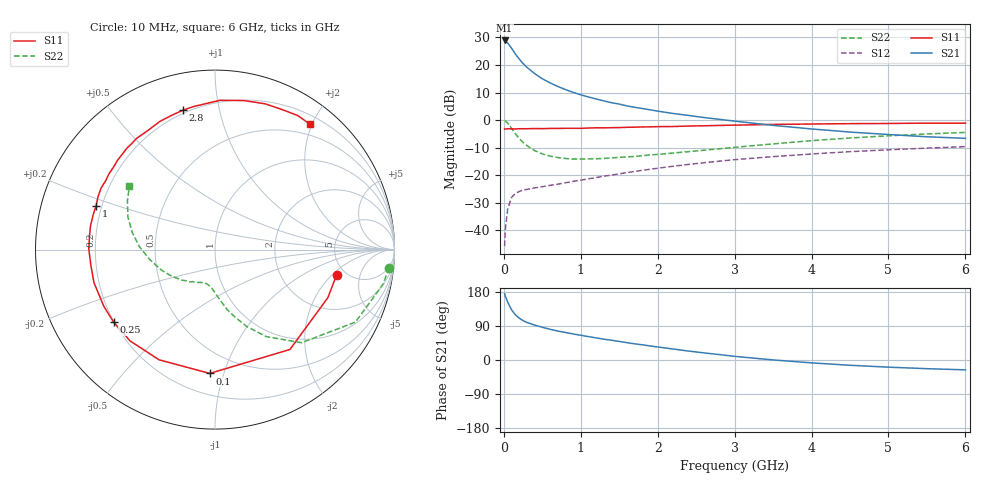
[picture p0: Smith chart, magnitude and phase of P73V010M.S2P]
! SIEMENS Small Signal Semiconductors
! BFP196
! Si NPN RF Bipolar Junction Transistor in SOT143
! VCE = 3 V  IC = 10 mA
! Common Emitter S-Parameters:  May  1996
# GHz  S  MA  R  50
!  f  S11  S21  S12  S22
! GHz  MAG  ANG  MAG  ANG  MAG  ANG  MAG  ANG
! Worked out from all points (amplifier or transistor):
!   36 points, 10 MHz to 6 GHz, reference 50 ohm
!   highest |S21| = 28.9 dB at 10 MHz (marker M1)
!   |S21| within 3 dB of that: start of sweep to 104.3 MHz
!   unconditionally stable (mu >= 1): 873 MHz to 3.271 GHz
!   at 250 MHz: K = 0.40, MSG = 23.0 dB, |S12| = -25.5 dB
!   at 1.4 GHz: K = 1.15, MAG = 10.8 dB, |S12| = -20.0 dB
!   at 6 GHz: K = 0.97, MSG = 1.5 dB, |S12| = -9.7 dB
!   S11 on the Smith chart (normalised r, x): 10 MHz: 4.22, -2.27; 100 MHz: 0.34, -0.90; 250 MHz: 0.20, -0.31; 1 GHz: 0.18, +0.17; 2.8 GHz: 0.18, +0.78; 6 GHz: 0.33, +1.97
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0.01  0.6923 -11.7  27.91 175.0  0.0051 87.7  0.9746 -6.0
0.02  0.6834 -23.1  27.28 168.0  0.0105 81.0  0.9564 -11.6
0.05  0.6956 -53.1  25.09 152.6  0.0242 66.6  0.8806 -27.3
0.1  0.6905 -92.4  20.18 132.6  0.0391 50.1  0.7083 -47.1
0.15  0.6885 -116.9  15.84 119.1  0.0463 41.6  0.5624 -59.5
0.2  0.6947 -132.9  12.89 110.4  0.0503 36.5  0.4632 -67.6
0.25  0.6943 -144.5  10.64 103.9  0.0531 33.9  0.3909 -73.6
0.3  0.6953 -152.9  9.083 99.1  0.0549 33.3  0.3436 -78.3
0.4  0.6991 -164.7  6.987 92.1  0.0584 33.1  0.2783 -84.8
0.5  0.6971 -173.0  5.625 86.3  0.0614 33.4  0.2426 -89.5
0.6  0.703 179.8  4.736 81.1  0.0649 35.3  0.2211 -93.6
0.7  0.7036 173.6  4.082 76.5  0.0683 36.9  0.2081 -97.5
0.8  0.706 169.2  3.576 72.6  0.0723 37.8  0.2002 -100.8
1  0.7061 159.7  2.873 65.2  0.0807 40.5  0.1953 -105.8
1.1  0.7155 155.6  2.618 61.7  0.0853 41.7  0.1963 -108.7
1.6  0.7367 137.5  1.805 45.7  0.1106 43.9  0.214 -122.6
2.2  0.7616 119.4  1.315 29.0  0.1445 42.2  0.2514 -137.4
2.8  0.7968 103.0  1.03 14.3  0.1787 37.7  0.2997 -153.9
3.5  0.8323 88.1  0.799 0.2  0.2162 30.4  0.3681 -171.4
4.5  0.859 71.0  0.604 -13.9  0.2662 19.5  0.4716 168.1
5.5  0.8778 58.3  0.496 -22.9  0.3087 8.1  0.5581 151.0
6  0.8767 52.8  0.465 -26.0  0.328 2.0  0.595 143.3
